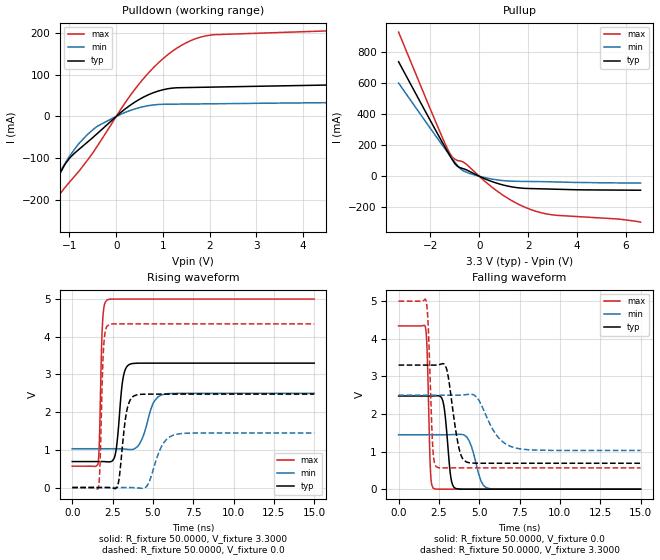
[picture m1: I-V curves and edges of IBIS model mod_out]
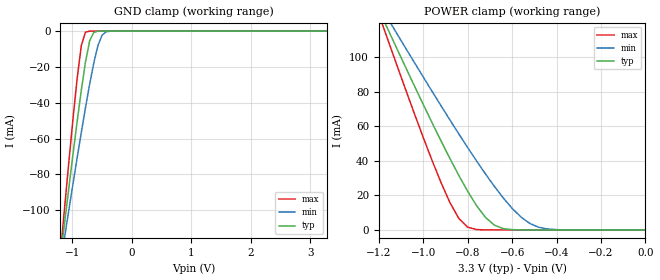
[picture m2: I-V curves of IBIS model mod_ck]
| IBIS (I/O, Buffer, Information, Specification) Model, officially
| electronic behavioral standard for Buffer structures of digital pins.
[IBIS ver]  4.0
[File name] rhfac2525.ibs
[File Rev]  1.0
[Date]   27 Nov 2015
[Source]   CAD & Design Services (Catania) - STMicroelectronics
[Notes]
  (Note1) This IBIS model assume Vcc=3.3V(TYP), 2.5V(MIN), 5.0V(MAX);
  (Note2) This IBIS model includes the Flat-14 package parasitic data;
[Copyright] (c) 2015 STMicroelectronics
|   Component RHFAC2525
[Component] RHFAC2525
[Manufacturer] STMicroelectronics
[Package]
| variable   typ   min   max
R_pkg   0.0   0.0   0.0
L_pkg   0.0H   0.0H   0.0H
C_pkg   0.0F   0.0F   0.0F
[Pin]  signal_name   model_name   R_pin   L_pin   C_pin
1   O0   mod_out   83.7m   2.67nH   1.03pF
2   O2   mod_out   28.3m   0.78nH   1.07pF
3   NC   NC   34.9m   0.88nH   0.82pF
4   GND   GND   34.9m   0.88nH   0.82pF
5   VCC   POWER   34.9m   0.88nH   0.82pF
6   O4   mod_out   28.3m   0.78nH   1.07pF
7   O6   mod_out   83.7m   2.67nH   1.03pF
8   O7   mod_out   83.7m   2.67nH   1.03pF
9   O5   mod_out   28.3m   0.78nH   1.07pF
10   GND   GND   34.9m   0.88nH   0.82pF
11   VCC   POWER   34.9m   0.88nH   0.82pF
12   CKIN   mod_ck   34.9m   0.88nH   0.82pF
13   O3   mod_out   28.3m   0.78nH   1.07pF
14   O1   mod_out   83.7m   2.67nH   1.03pF
| Models and submodels in the file (2): mod_out (Output), mod_ck (Input)
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|   Model mod_out
[Model]   mod_out
Model_type Output
|Vinl  =   1.000V
|Vinh  =   2.300V
Vmeas =   1.650V
Cref  =   50pF
Rref  =   500
C_comp   11.120pF   10.144pF   11.640pF
[Temperature Range]  25.0000   0.1250k   -55.0000
[Voltage Range]   3.3000V   2.5000V   5.0000V
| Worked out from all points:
|   slope of the pulldown table from 0 to 0.495 V, typ, clamps not added: 12.1 ohm
|   slope of the pullup table from 0 to 0.495 V, typ, clamps not added: 15.1 ohm
|   rising waveform, R_fixture 50.0000, V_fixture 3.3000: 20-80 % time 324ps typ, 630ps min, 153ps max; typ from 0.689 V to 3.3 V
|   rising waveform, R_fixture 50.0000, V_fixture 0.0: 20-80 % time 382ps typ, 742ps min, 174ps max; typ from 0 V to 2.48 V
|   falling waveform, R_fixture 50.0000, V_fixture 0.0: 20-80 % time 306ps typ, 558ps min, 157ps max; typ from 2.48 V to 0 V
|   falling waveform, R_fixture 50.0000, V_fixture 3.3000: 20-80 % time 531ps typ, 1.13ns min, 220ps max; typ from 3.3 V to 0.689 V
[Pulldown]
|Voltage   I(typ)   I(min)   I(max)
-3.3V     -735.2mA   -598mA     -926.2mA
-1.9V     -328.4mA   -284.8mA   -393.4mA
-1.7V     -271.2mA   -240.6mA   -319.1mA
-1.6V     -242.8mA   -218.7mA   -282.5mA
-1.1V     -115.8mA   -113.4mA   -171.3mA
-800mV    -79.37mA   -65.42mA   -132mA
-400mV    -40.59mA   -23.29mA   -70.55mA
600mV     47.46mA    24.08mA    93.18mA
1.1V      66.62mA    29.5mA     148.2mA
1.6V      69.76mA    30.04mA    182.8mA
2.1V      70.78mA    30.59mA    196.8mA
6.6V      79.84mA    35.34mA    215.3mA
[Pullup]
|Voltage   I(typ)   I(min)   I(max)
-3.3V     736.1mA    598.9mA    926.9mA
-1.5V     214.8mA    197.5mA    245.7mA
-1.2V     131.8mA    132.8mA    145.8mA
-1V       81.28mA    91.02mA    110mA
-900mV    64.69mA    71.04mA    101.6mA
-700mV    50.85mA    39.04mA    94.89mA
100mV     -7.313mA   -4.002mA   -14.37mA
1.2V      -64.28mA   -30.68mA   -144.7mA
2.2V      -79.5mA    -33.87mA   -219mA
3.1V      -83.22mA   -36.47mA   -250.1mA
5.6V      -88.81mA   -42.63mA   -274.1mA
6.6V      -89.81mA   -43.66mA   -295.3mA
[Ramp]
| variable   typ   min   max
dV/dt_r   1.4869/0.4172n   0.8687/0.7930n   2.6051/0.2194n
dV/dt_f   1.5671/0.5504n   0.8827/1.1360n   2.6607/0.2370n
R_load = 50.0000
[Rising Waveform]
R_fixture= 50.0000
V_fixture= 3.3000
V_fixture_min= 2.5000
V_fixture_max= 5.0000
|time   V(typ)   V(min)   V(max)
0s        688.9mV    1.029V     566mV
1.59ns    689.1mV    1.029V     609.7mV
1.68ns    689.2mV    1.029V     1.218V
1.875ns   688.7mV    1.029V     4.358V
2.175ns   682.1mV    1.029V     4.982V
2.655ns   855mV      1.03V      5V
3.135ns   2.864V     1.024V     5V
3.585ns   3.274V     1.007V     5V
5.505ns   3.3V       2.453V     5V
15ns      3.3V       2.5V       5V
[Rising Waveform]
R_fixture= 50.0000
V_fixture= 0.0
V_fixture_min= 0.0
V_fixture_max= 0.0
|time   V(typ)   V(min)   V(max)
0s        127pV      42.74nV    100pV
1.605ns   -17.06uV   -907.4nV   -27.43mV
1.725ns   44.43uV    -4.214uV   653.2mV
1.965ns   497.5uV    -11.44uV   3.847V
2.295ns   -1.562mV   -12.39uV   4.329V
2.865ns   133.5mV    182.1uV    4.342V
3.345ns   1.955V     575uV      4.342V
3.825ns   2.43V      -3.692mV   4.342V
6.255ns   2.478V     1.387V     4.342V
15ns      2.478V     1.448V     4.342V
[Falling Waveform]
R_fixture= 50.0000
V_fixture= 0.0
V_fixture_min= 0.0
V_fixture_max= 0.0
|time   V(typ)   V(min)   V(max)
0s        2.478V     1.448V     4.342V
1.65ns    2.478V     1.448V     4.335V
1.755ns   2.478V     1.448V     3.819V
1.965ns   2.478V     1.448V     576mV
2.145ns   2.479V     1.448V     23.01mV
2.745ns   2.344V     1.447V     33.03uV
3.225ns   350.9mV    1.449V     599.7nV
3.48ns    31.65mV    1.453V     61.07nV
5.565ns   497.8nV    21.68mV    -12.8nV
15ns      -3.603nV   33.47nV    -12.8nV
[Falling Waveform]
R_fixture= 50.0000
V_fixture= 3.3000
V_fixture_min= 2.5000
V_fixture_max= 5.0000
|time   V(typ)   V(min)   V(max)
0s        3.3V       2.5V       5V
1.695ns   3.3V       2.5V       5.024V
1.845ns   3.3V       2.5V       4.249V
2.115ns   3.299V     2.5V       1.131V
2.325ns   3.3V       2.5V       598.3mV
2.955ns   3.225V     2.5V       566mV
3.735ns   1.104V     2.5V       566mV
4.215ns   721.1mV    2.516V     566mV
7.065ns   688.9mV    1.119V     566mV
15ns      688.9mV    1.029V     566mV
|   Model mod_ck
[Model]   mod_ck
Model_type Input
Vinl  =   1.000V
Vinh  =   2.300V
C_comp   2.119pF   2.024pF   2.219pF
[Model Spec]
|hysteresis   (deltaV = 50mV)
Vinh+   1.680V   NA   NA
Vinh-   1.670V   NA   NA
Vinl+   1.630V   NA   NA
Vinl-   1.620V   NA   NA
[Temperature Range]  25.0000   0.1250k   -55.0000
[Voltage Range]   3.3000V   2.5000V   5.0000V
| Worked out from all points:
|   GND clamp passes 1 mA (typ) near -0.64 V on its own axis
|   POWER clamp passes 1 mA (typ) near -0.64 V on its own axis
[GND_clamp]
|Voltage   I(typ)   I(min)   I(max)
-3.3V     -734.4mA   -597.5mA   -923.2mA
-1.2V     -126.4mA   -130mA     -123.9mA
-1.13V    -107mA     -115mA     -98.44mA
-1.06V    -87.81mA   -100.1mA   -73.44mA
-920mV    -50.6mA    -70.84mA   -26.61mA
-850mV    -33.12mA   -56.62mA   -8.161mA
-780mV    -17.36mA   -42.84mA   -579.9uA
-710mV    -5.491mA   -29.73mA   -15.45uA
-640mV    -698.4uA   -17.8mA    -374.1nA
-500mV    -3.363uA   -2.251mA   -230.1pA
-430mV    -220.7nA   -381uA     -16.99pA
3.28V     6.535pA    11.74uA    3.12pA
[POWER_clamp]
|Voltage   I(typ)   I(min)   I(max)
-3.28V    729.5mA    594mA      916.5mA
-1.2V     127.4mA    131mA      124.8mA
-1.16V    116.3mA    122.4mA    110.2mA
-1.12V    105.2mA    113.8mA    95.75mA
-920mV    51.49mA    71.8mA     27.39mA
-840mV    31.56mA    55.55mA    6.701mA
-800mV    22.36mA    47.63mA    1.624mA
-720mV    7.281mA    32.4mA     29.18uA
-680mV    2.795mA    25.23mA    3.489uA
-520mV    8.135uA    3.753mA    714.2pA
-400mV    76.29nA    182.9uA    12.79pA
0V        6.622pA    2.124nA    10pA
